PROGRAM MAIN_CM
VAR CONSTANT										
	cInitPowerCep 	: ST_CM_PowerCepstrum_InitPars  := (	nFFT_Length    := cFFTLength, 
												    	    nWindowLength  := cWindowLength);		

	cInitPowerSpectrum : ST_CM_PowerSpectrum_InitPars := (	nFFT_Length    := cFFTLength, 
												    	    nWindowLength  := cWindowLength);												
END_VAR

VAR												
	fbPowerCepstrum	: FB_CMA_PowerCepstrum :=(	stInitPars := cInitPowerCep, 
												nOwnID := eID_PowerCepstrum, 
												aDestIDs := [eID_Sink_Ceps] );		

	fbPowerSpectrum	: FB_CMA_PowerSpectrum :=(	stInitPars := cInitPowerSpectrum, 
												nOwnID := eID_PowerSpectrum, 
												aDestIDs := [eID_Sink_Spec] );													
	
	fbErrHist			: FB_HRErrHist; // error monitoring
END_VAR


// Call fbPowerCepstrum 
fbPowerCepstrum.Call();
IF fbPowerCepstrum.bError THEN
	fbErrHist.AddError(bErr:=TRUE, hrErrCode:=fbPowerCepstrum.hrErrorCode, sErrSource:='MAIN_CM.fbPowerCepstrum'); // error monitoring
	// ToDo: if error
END_IF

// Call fbPowerSpectrum
fbPowerSpectrum.Call();
IF fbPowerSpectrum.bError THEN
	fbErrHist.AddError(bErr:=TRUE, hrErrCode:=fbPowerSpectrum.hrErrorCode, sErrSource:='MAIN_CM.fbPowerSpectrum'); // error monitoring
	// ToDo: if error
END_IF

END_PROGRAM
